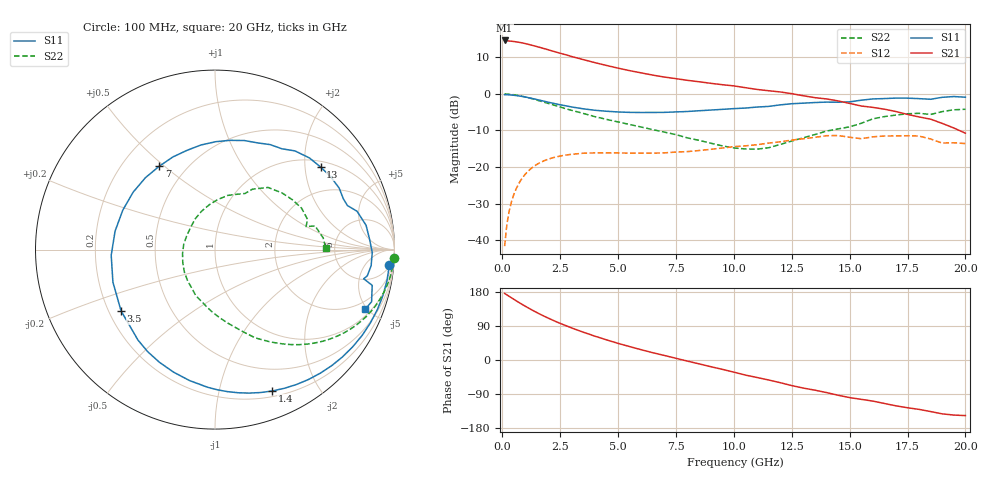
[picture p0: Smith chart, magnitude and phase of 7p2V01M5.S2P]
! Infineon Technologies  Discrete & RF Semiconductors
! bfp620
! VCE =  2.0 V,  IC =  1.5 mA
! Common Emitter S-Parameters:  Sep 2002
# GHz  S  MA  R  50
!  f  S11  S21  S12  S22
! GHz  MAG  ANG  MAG  ANG  MAG  ANG  MAG  ANG
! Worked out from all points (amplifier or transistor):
!   59 points, 100 MHz to 20 GHz, reference 50 ohm
!   highest |S21| = 14.6 dB at 100 MHz (marker M1)
!   |S21| within 3 dB of that: start of sweep to 2.227 GHz
!   unconditionally stable (mu >= 1): 6.028 GHz to 15.7 GHz; 17.73 GHz to end of sweep
!   at 1 GHz: K = 0.13, MSG = 17.8 dB, |S12| = -21.9 dB
!   at 5.5 GHz: K = 0.91, MSG = 11.3 dB, |S12| = -16.2 dB
!   at 20 GHz: K = 1.34, MAG = -2.1 dB, |S12| = -13.6 dB
!   S11 on the Smith chart (normalised r, x): 100 MHz: 6, -20; 1.4 GHz: 0.26, -1.45; 3.5 GHz: 0.25, -0.28; 7 GHz: 0.36, +0.48; 13 GHz: 1.16, +2.42; 20 GHz: 1.38, -4.84
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0.1  0.9749 -5.2  5.37 175.6  0.0083 81.2  0.9984 -2.8
0.3  0.9701 -15.2  5.278 167.9  0.0253 81.4  0.9888 -8.4
0.5  0.9573 -25.3  5.193 160.1  0.0424 75.6  0.9723 -13.8
0.8  0.9285 -40.1  5.015 148.8  0.0662 66.2  0.936 -21.4
1.1  0.8915 -54.3  4.776 138.2  0.0869 57.3  0.8897 -28.5
1.4  0.85 -67.9  4.513 128.2  0.104 49.2  0.8385 -34.8
1.9  0.781 -89.1  4.076 112.9  0.1253 37.5  0.7536 -43.9
2.4  0.7207 -108.7  3.666 99.2  0.1393 27.8  0.6761 -51.5
3  0.662 -130.4  3.237 84.5  0.1494 18.0  0.5953 -59.5
3.5  0.6249 -146.9  2.938 73.3  0.1547 11.2  0.5405 -65.5
4  0.597 -162.3  2.672 62.9  0.1561 5.1  0.4883 -70.6
5  0.5661 169.5  2.248 43.9  0.1559 -3.2  0.414 -80.4
6  0.5571 145.0  1.936 27.1  0.1551 -8.9  0.3526 -91.6
7  0.5587 123.8  1.698 12.0  0.1563 -12.3  0.3002 -104.0
9  0.6012 89.6  1.395 -17.6  0.1747 -18.8  0.212 -143.4
10.5  0.64 68.3  1.215 -39.8  0.1949 -27.0  0.1768 170.5
12  0.7076 51.0  1.063 -59.8  0.2213 -34.8  0.2036 122.9
13  0.747 38.0  0.942 -74.1  0.2439 -42.9  0.2511 97.6
13.5  0.7617 32.2  0.888 -79.6  0.2548 -47.5  0.278 87.3
15  0.7776 18.4  0.741 -99.2  0.2553 -67.2  0.3544 61.9
17  0.8763 -1.0  0.574 -120.9  0.2662 -81.0  0.5135 32.6
20  0.9001 -21.7  0.29 -146.7  0.2095 -106.0  0.6163 1.0
